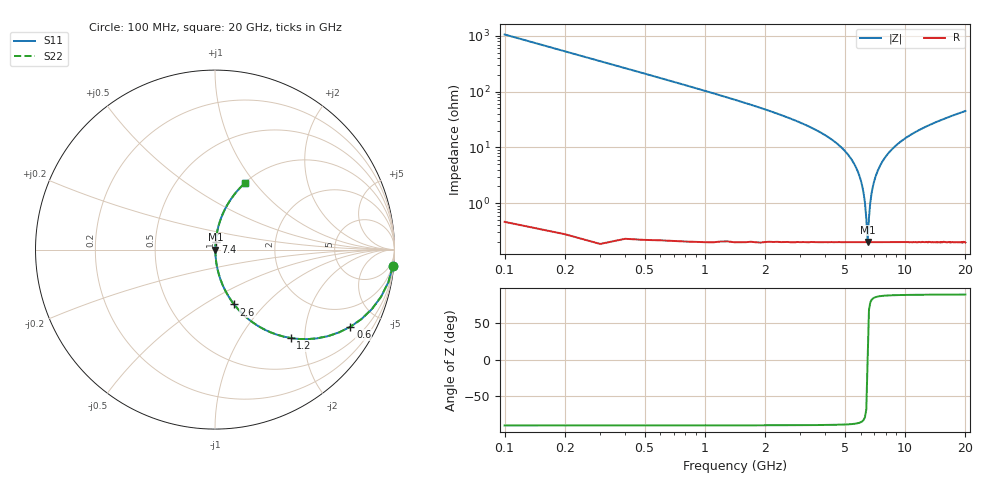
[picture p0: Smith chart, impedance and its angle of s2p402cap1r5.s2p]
! AVX Thin Film Operation		Date: April 2003
! Description: Accu-P® Series, Thin Film, SMD, RF Capacitor
! Part Number: 04021J1R5ABS
! 50 MHz  -  20 GHz
! Serial Measurements
# hz S db R 50
!	S11		S21		S12		S22
!	dB	Phase	dB	Phase	dB	Phase	dB	Phase
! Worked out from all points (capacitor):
!   200 points, 100 MHz to 20 GHz, reference 50 ohm
!   read as one part in series: C = 1.5 pF near 200 MHz
!   lowest |Z| = 200 mohm at 6.5 GHz (marker M1)
!   series resonance near 6.497 GHz, so ESL is about 400 pH
!   S11 on the Smith chart (normalised r, x): 100 MHz: 1, -21; 600 MHz: 1.00, -3.51; 1.2 GHz: 1.00, -1.71; 2.6 GHz: 1.00, -0.69; 7.4 GHz: 1.00, +0.09; 20 GHz: 1.00, +0.90
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1e8  -0.04 -5.4  -20.55 84.6  -20.55 84.6  -0.04 -5.4
2e8  -0.15 -10.7  -14.64 79.3  -14.64 79.3  -0.15 -10.7
3e8  -0.34 -15.8  -11.29 74.2  -11.29 74.2  -0.34 -15.8
6e8  -1.23 -29.7  -6.11 60.2  -6.11 60.2  -1.23 -29.7
1.2e9  -3.76 -49.4  -2.39 40.4  -2.39 40.4  -3.76 -49.4
2.6e9  -9.80 -70.8  -0.50 18.9  -0.50 18.9  -9.80 -70.8
3.5e9  -13.56 -77.3  -0.21 12.1  -0.21 12.1  -13.56 -77.3
5e9  -21.30 -83.7  -0.05 4.9  -0.05 4.9  -21.30 -83.7
5.8e9  -28.61 -84.8  -0.02 2.1  -0.02 2.1  -28.61 -84.8
6.1e9  -33.69 -83.3  -0.02 1.2  -0.02 1.2  -33.69 -83.3
6.3e9  -39.78 -78.2  -0.02 0.6  -0.02 0.6  -39.78 -78.2
6.4e9  -45.49 -67.7  -0.02 0.3  -0.02 0.3  -45.49 -67.7
6.5e9  -53.98 3.6  -0.02 -0.0  -0.02 -0.0  -53.98 3.6
6.6e9  -45.22 68.3  -0.02 -0.3  -0.02 -0.3  -45.22 68.3
6.8e9  -36.50 81.5  -0.02 -0.9  -0.02 -0.9  -36.50 81.5
7e9  -32.26 83.9  -0.02 -1.4  -0.02 -1.4  -32.26 83.9
7.4e9  -27.43 84.9  -0.03 -2.4  -0.03 -2.4  -27.43 84.9
8.5e9  -21.08 83.7  -0.05 -5.1  -0.05 -5.1  -21.08 83.7
1.01e10  -16.66 80.8  -0.11 -8.4  -0.11 -8.4  -16.66 80.8
1.34e10  -12.08 75.1  -0.30 -14.4  -0.30 -14.4  -12.08 75.1
1.67e10  -9.50 70.1  -0.53 -19.6  -0.53 -19.6  -9.50 70.1
2e10  -7.76 65.6  -0.81 -24.2  -0.81 -24.2  -7.76 65.6
